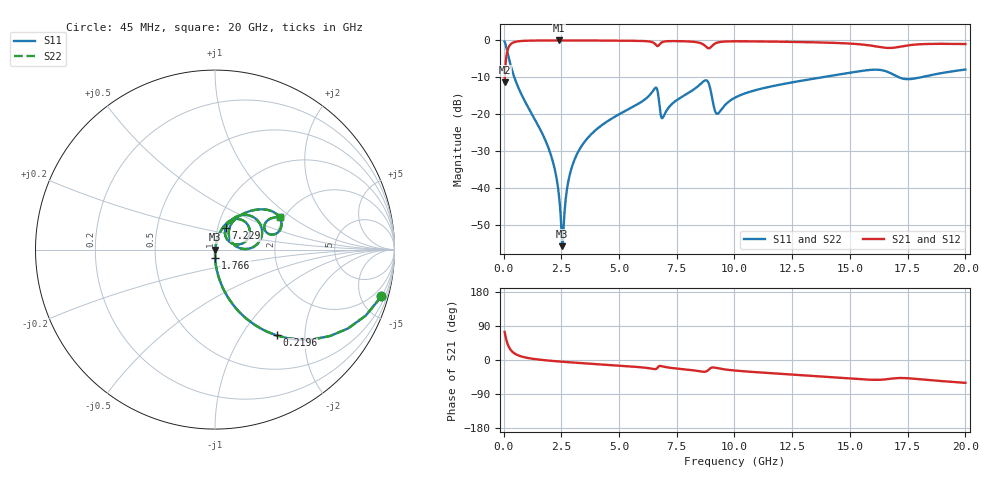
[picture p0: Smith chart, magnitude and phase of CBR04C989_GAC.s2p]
! S-parameter model data by Modelithics Inc.  support@modelithics.com 813-866-6335  Tampa FL USA
! S-Parameter data specifications:
! Substrate: 20-mil Rogers 4350B, substrate thickness, H=0.508mm, Dielectric constant, Er=3.75
! PCB Mounting Pad Footprint: Pad width, PadW=0.52mm , Pad length, PadL=0.52mm , Pad gap, PadG (edge-to-edge)=0.28mm , Reference planes=1.32mm apart
#  GHz  S  MA  R 50
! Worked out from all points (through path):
!   801 points, 45 MHz to 20 GHz, reference 50 ohm
!   highest |S21| = -0.01 dB at 2.415 GHz (marker M1); lowest = -11.4 dB at 45 MHz (marker M2)
!   group delay of S21, straight-line fit = 9.63 ps
!   lowest |S11| = -55.7 dB at 2.539 GHz (marker M3), VSWR 1.00, Z = 50.2 - j0.066 ohm
!   |S11| at or under -10 dB: 466.9 MHz to 13.78 GHz (13.31 GHz wide, 187 % of centre); 17.12 GHz to 18.06 GHz (941.1 MHz wide, 5.35 % of centre)
!   |S22| runs from -55.7 to -0.3 dB; largest |S21 - S12| = 0
!   S11 on the Smith chart (normalised r, x): 45 MHz: 0.99, -7.12; 219.6 MHz: 0.99, -1.45; 1.766 GHz: 1.00, -0.10; 7.229 GHz: 1.09, +0.26; 20 GHz: 1.90, +0.82
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0.045  0.9631 -15.7  0.2692 74.3  0.2692 74.3  0.9631 -15.7
0.219606  0.5883 -54.3  0.8082 35.6  0.8082 35.6  0.5883 -54.3
0.593762  0.2485 -76.5  0.9679 13.3  0.9679 13.3  0.2485 -76.5
1.766119  0.04771 -89.0  0.9975 -0.5  0.9975 -0.5  0.04771 -89.0
2.190163  0.01954 -88.7  0.9983 -2.9  0.9983 -2.9  0.01954 -88.7
2.414656  0.007145 -81.8  0.9984 -4.0  0.9984 -4.0  0.007145 -81.8
2.539375  0.001637 -23.7  0.9984 -4.6  0.9984 -4.6  0.001637 -23.7
2.614206  0.003557 58.8  0.9983 -4.9  0.9983 -4.9  0.003557 58.8
2.738925  0.009338 74.5  0.9983 -5.5  0.9983 -5.5  0.009338 74.5
2.888587  0.0162 77.9  0.9981 -6.2  0.9981 -6.2  0.0162 77.9
3.387462  0.03748 78.9  0.9974 -8.3  0.9974 -8.3  0.03748 78.9
6.530375  0.2203 49.5  0.9151 -24.1  0.9151 -24.1  0.2203 49.5
6.704981  0.1763 14.8  0.8465 -17.6  0.8465 -17.6  0.1763 14.8
6.879588  0.08863 41.1  0.9498 -16.8  0.9498 -16.8  0.08863 41.1
7.2288  0.1319 63.7  0.9781 -20.7  0.9781 -20.7  0.1319 63.7
8.725425  0.287 34.7  0.8467 -31.0  0.8467 -31.0  0.287 34.7
9.249244  0.1014 29.4  0.9324 -21.3  0.9324 -21.3  0.1014 29.4
10.0225  0.1679 57.6  0.9722 -27.8  0.9722 -27.8  0.1679 57.6
13.36496  0.301 46.4  0.9437 -41.8  0.9437 -41.8  0.301 46.4
16.68248  0.3693 15.8  0.7896 -50.0  0.7896 -50.0  0.3693 15.8
17.55551  0.2987 22.4  0.8601 -48.3  0.8601 -48.3  0.2987 22.4
20  0.4034 26.6  0.8926 -60.3  0.8926 -60.3  0.4034 26.6
